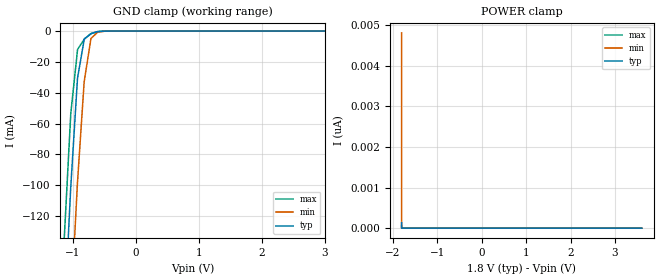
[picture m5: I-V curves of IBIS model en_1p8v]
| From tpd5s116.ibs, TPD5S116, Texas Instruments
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[Model]   en_1p8v
Model_type   Input
Vinl = 0.4
Vinh = 1
|   typ   min   max
|   (nom PVT)   (slow PVT)   (fast PVT)
C_comp   0.787p   0.739p   0.858p
| Where nom  PVT is Nominal Process, 1.8V, 27C
|   Fast PVT is Strong Process,  2.0V, -40C
|   Slow PVT is Weak Process,   1.6V, 125C
[Voltage Range]   1.8   1.6   2
[Temperature Range]   27   125   -40
[Power Clamp Reference]   1.8   1.6   2
[GND Clamp Reference]   -0   -0   -0
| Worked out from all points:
|   GND clamp passes 1 mA (typ) near -0.67 V on its own axis
[GND Clamp]
|   Voltage   I(typ)   I(min)   I(max)
-1.8V     -807.1mA   -888.9mA   -756.2mA
-1.144V   -190.6mA   -274.9mA   -137.6mA
-1.039V   -103.3mA   -184.5mA   -55.81mA
-1.036V   -100.9mA   -182mA     -53.38mA
-930.7mV  -31.82mA   -99.22mA   -13.08mA
-928.9mV  -30.6mA    -98.08mA   -12.37mA
-927.6mV  -30.3mA    -97.3mA    -11.89mA
-822.7mV  -5.547mA   -32.79mA   -5.341mA
-712.9mV  -1.526mA   -4.704mA   -1.711mA
-606.7mV  -347.3uA   -685.6uA   -302.2uA
-498.7mV  -45.92uA   -112.7uA   -29.06uA
3.6V      0A         0A         0A
[POWER Clamp]
|   Voltage   I(typ)   I(min)   I(max)
-1.8V     138.9pA    4.805nA    68.47pA
-1.8V     0A         0A         0A
-1.8V     0A         0A         0A
3.6V      0A         0A         0A
